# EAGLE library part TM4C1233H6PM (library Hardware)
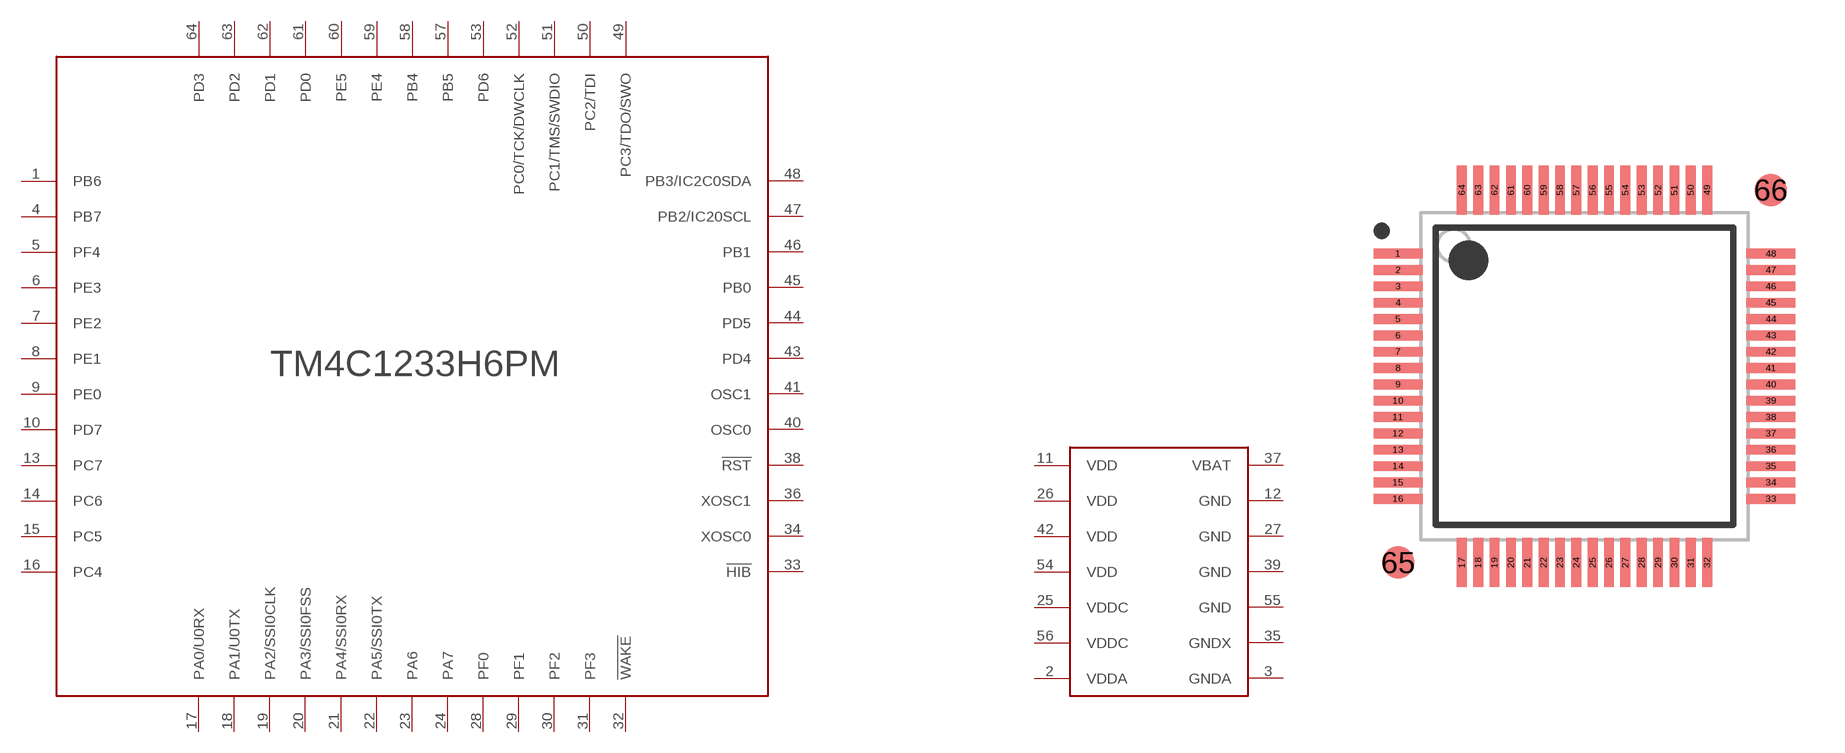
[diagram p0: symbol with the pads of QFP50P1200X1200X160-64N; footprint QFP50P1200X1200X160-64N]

Designator prefix -; gates G$1=TM4C1233H6PM_UC G$2=TM4C1233H6PM_PWR

## TM4C1233H6PM  [QFP50P1200X1200X160-64N]
1  G$1:PB6
2  G$2:VDDA
3  G$2:GNDA
4  G$1:PB7
5  G$1:PF4
6  G$1:PE3
7  G$1:PE2
8  G$1:PE1
9  G$1:PE0
10  G$1:PD7
11  G$2:VDD
12  G$2:GND
13  G$1:PC7
14  G$1:PC6
15  G$1:PC5
16  G$1:PC4
17  G$1:PA0/U0RX
18  G$1:PA1/U0TX
19  G$1:PA2/SSI0CLK
20  G$1:PA3/SSI0FSS
21  G$1:PA4/SSI0RX
22  G$1:PA5/SSI0TX
23  G$1:PA6
24  G$1:PA7
25  G$2:VDDC
26  G$2:VDD
27  G$2:GND
28  G$1:PF0
29  G$1:PF1
30  G$1:PF2
31  G$1:PF3
32  G$1:!WAKE
33  G$1:!HIB
34  G$1:XOSC0
35  G$2:GNDX
36  G$1:XOSC1
37  G$2:VBAT
38  G$1:!RST
39  G$2:GND
40  G$1:OSC0
41  G$1:OSC1
42  G$2:VDD
43  G$1:PD4
44  G$1:PD5
45  G$1:PB0
46  G$1:PB1
47  G$1:PB2/IC20SCL
48  G$1:PB3/IC2C0SDA
49  G$1:PC3/TDO/SWO
50  G$1:PC2/TDI
51  G$1:PC1/TMS/SWDIO
52  G$1:PC0/TCK/DWCLK
53  G$1:PD6
54  G$2:VDD
55  G$2:GND
56  G$2:VDDC
57  G$1:PB5
58  G$1:PB4
59  G$1:PE4
60  G$1:PE5
61  G$1:PD0
62  G$1:PD1
63  G$1:PD2
64  G$1:PD3

## Footprint QFP50P1200X1200X160-64N (pad centres in mm)
PCB Libraries Package
smd 1.5 x 0.3: 1 -5.7,3.75; 2 -5.7,3.25; 3 -5.7,2.75; 4 -5.7,2.25; 5 -5.7,1.75; 6 -5.7,1.25; 7 -5.7,0.75; 8 -5.7,0.25; 9 -5.7,-0.25; 10 -5.7,-0.75; 11 -5.7,-1.25; 12 -5.7,-1.75; 13 -5.7,-2.25; 14 -5.7,-2.75; 15 -5.7,-3.25; 16 -5.7,-3.75; 33 5.7,-3.75; 34 5.7,-3.25; 35 5.7,-2.75; 36 5.7,-2.25; 37 5.7,-1.75; 38 5.7,-1.25; 39 5.7,-0.75; 40 5.7,-0.25; 41 5.7,0.25; 42 5.7,0.75; 43 5.7,1.25; 44 5.7,1.75; 45 5.7,2.25; 46 5.7,2.75; 47 5.7,3.25; 48 5.7,3.75
smd 0.3 x 1.5: 17 -3.75,-5.7; 18 -3.25,-5.7; 19 -2.75,-5.7; 20 -2.25,-5.7; 21 -1.75,-5.7; 22 -1.25,-5.7; 23 -0.75,-5.7; 24 -0.25,-5.7; 25 0.25,-5.7; 26 0.75,-5.7; 27 1.25,-5.7; 28 1.75,-5.7; 29 2.25,-5.7; 30 2.75,-5.7; 31 3.25,-5.7; 32 3.75,-5.7; 49 3.75,5.7; 50 3.25,5.7; 51 2.75,5.7; 52 2.25,5.7; 53 1.75,5.7; 54 1.25,5.7; 55 0.75,5.7; 56 0.25,5.7; 57 -0.25,5.7; 58 -0.75,5.7; 59 -1.25,5.7; 60 -1.75,5.7; 61 -2.25,5.7; 62 -2.75,5.7; 63 -3.25,5.7; 64 -3.75,5.7
smd 1 x 1: 65 -5.7,-5.7; 66 5.7,5.7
